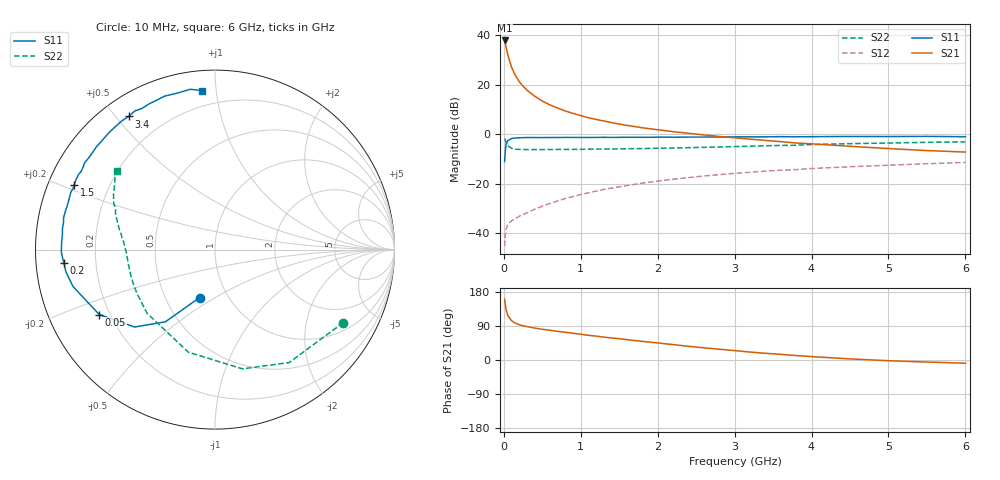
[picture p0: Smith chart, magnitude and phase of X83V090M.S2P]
! SIEMENS Small Signal Semiconductors
! BFP136W
! Si NPN RF Bipolar Junction Transistor in SOT343
! VCE = 3 V  IC = 90 mA
! Common Emitter S-Parameters:  September  1994
# GHz  S  MA  R  50
!  f  S11  S21  S12  S22
! GHz  MAG  ANG  MAG  ANG  MAG  ANG  MAG  ANG
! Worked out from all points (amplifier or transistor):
!   40 points, 10 MHz to 6 GHz, reference 50 ohm
!   highest |S21| = 37.8 dB at 10 MHz (marker M1)
!   |S21| within 3 dB of that: start of sweep to 31.79 MHz
!   unconditionally stable (mu >= 1): 516.2 MHz to 2.954 GHz
!   at 200 MHz: K = 0.67, MSG = 27.2 dB, |S12| = -33.1 dB
!   at 1.5 GHz: K = 1.10, MAG = 10.7 dB, |S12| = -21.2 dB
!   at 6 GHz: K = 0.97, MSG = 2.1 dB, |S12| = -11.4 dB
!   S11 on the Smith chart (normalised r, x): 10 MHz: 0.74, -0.43; 50 MHz: 0.16, -0.26; 200 MHz: 0.08, -0.05; 1.5 GHz: 0.08, +0.22; 3.4 GHz: 0.08, +0.54; 6 GHz: 0.11, +0.92
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0.01  0.2802 -107.7  77.91 160.5  0.0055 69.9  0.8226 -29.6
0.02  0.4882 -124.5  67.04 144.2  0.0096 57.0  0.753 -56.7
0.03  0.622 -136.1  56.84 132.5  0.0123 49.5  0.682 -77.0
0.05  0.7392 -150.7  40.65 118.3  0.015 40.2  0.5905 -104.6
0.1  0.8173 -165.4  22.54 103.6  0.0178 35.3  0.5187 -136.8
0.15  0.8399 -171.5  15.33 97.2  0.0198 39.1  0.499 -150.3
0.2  0.8447 -174.8  11.52 93.2  0.0221 41.2  0.493 -157.6
0.25  0.8527 -177.7  9.286 90.3  0.0241 44.6  0.4912 -162.3
0.3  0.8563 -179.4  7.769 88.2  0.0258 46.8  0.4892 -165.4
0.4  0.8555 176.9  5.854 84.3  0.0306 51.3  0.4892 -169.6
0.5  0.8544 174.3  4.665 81.0  0.0352 54.1  0.4896 -172.4
0.6  0.858 172.2  3.891 78.5  0.04 56.9  0.4907 -174.3
0.7  0.8572 169.9  3.358 75.5  0.045 58.6  0.4918 -175.7
0.9  0.8607 166.2  2.625 70.5  0.0551 60.1  0.4942 -178.2
1.1  0.8591 162.0  2.149 65.1  0.0658 60.9  0.4976 -179.9
1.5  0.864 155.2  1.601 56.1  0.0869 60.2  0.505 177.0
2.2  0.8693 143.0  1.126 40.6  0.1232 55.4  0.5258 171.6
3.2  0.8851 126.1  0.794 21.0  0.1705 46.0  0.5717 162.9
3.4  0.8847 123.0  0.75 17.7  0.1802 43.8  0.585 161.1
4.5  0.8999 108.0  0.57 2.9  0.2203 33.6  0.6446 151.3
5.5  0.9037 98.8  0.467 -5.4  0.2535 25.8  0.6848 144.5
6  0.8887 94.5  0.436 -8.4  0.2697 21.3  0.7001 141.5
